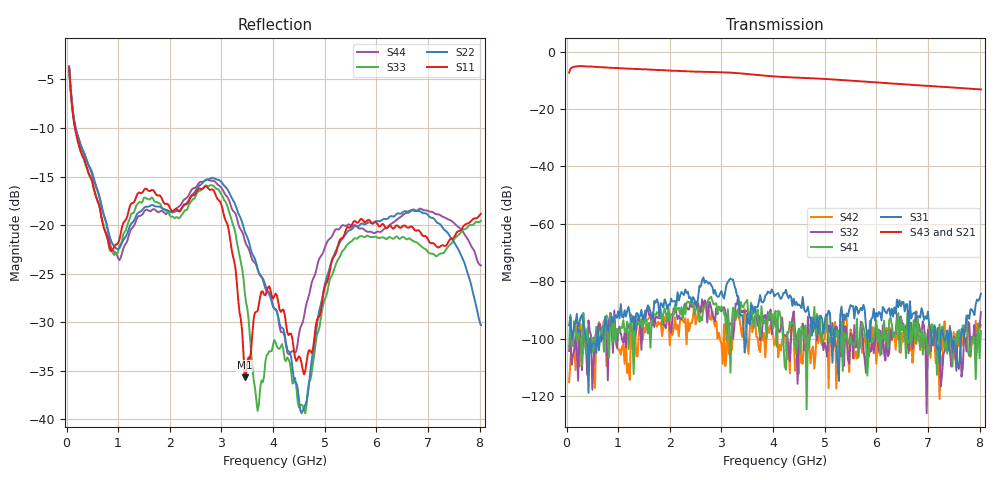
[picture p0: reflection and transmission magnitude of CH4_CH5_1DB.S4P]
!Agilent Technologies,E5071C,MY46316741,A.11.02
!Date: Mon Jun 01 11:48:19 2026
!Data & Calibration Information:
!1:CH4 INPUT 2:CH4 OUTPUT 3:CH5 INPUT 4:CH5 OUTPUT
!Freq	S11:SOLT4(ON)	S12:SOLT4(ON)	S13:SOLT4(ON)	S14:SOLT4(ON)
!	S21:SOLT4(ON)	S22:SOLT4(ON)	S23:SOLT4(ON)	S24:SOLT4(ON)
!	S31:SOLT4(ON)	S32:SOLT4(ON)	S33:SOLT4(ON)	S34:SOLT4(ON)
!	S41:SOLT4(ON)	S42:SOLT4(ON)	S43:SOLT4(ON)	S44:SOLT4(ON)
!PortZ  Port1:50+j0  Port2:50+j0  Port3:50+j0  Port4:50+j0
!Above PortZ is port z conversion or system Z0 setting when saving the data.
!When reading, reference impedance value at option line is always used.
# Hz S dB R 50
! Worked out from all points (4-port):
!   320 points, 50 MHz to 8.025 GHz, reference 50 ohm
!   strongest paths, dB at 50 MHz, 2.05 GHz, 4.05 GHz, 6.05 GHz, 8.025 GHz:
!     S43: -7.3, -6.7, -8.7, -10.8, -13.2
!     S21: -7.4, -6.8, -8.9, -11.0, -13.4
!     S31: -95.3, -87.0, -84.7, -90.6, -84.3
!     S41: -102.9, -91.8, -90.2, -96.7, -97.3
!     S32: -104.2, -93.2, -96.0, -104.2, -90.7
!     S42: -115.0, -98.7, -100.5, -104.8, -95.2
!   lowest |S11| = -35.7 dB at 3.45 GHz (marker M1), VSWR 1.03, Z = 49.1 - j1.38 ohm
!   |S11| at or under -10 dB: 164.9 MHz to end of sweep
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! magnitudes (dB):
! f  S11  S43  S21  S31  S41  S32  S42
! 50 MHz  -3.8  -7.3  -7.4  -95.3  -102.9  -104.2  -115.0
! 1.025 GHz  -21.5  -5.8  -6.0  -92.9  -97.9  -95.7  -103.7
! 2.85 GHz  -16.4  -7.2  -7.3  -84.3  -88.1  -92.9  -93.8
! 3.45 GHz  -35.7  -7.7  -7.9  -104.8  -87.6  -90.9  -89.7
! 4.55 GHz  -34.2  -9.2  -9.4  -89.3  -95.7  -98.3  -108.4
! 5.575 GHz  -19.6  -10.2  -10.4  -92.9  -102.4  -95.2  -106.8
! 8.025 GHz  -18.8  -13.2  -13.4  -84.3  -97.3  -90.7  -95.2
